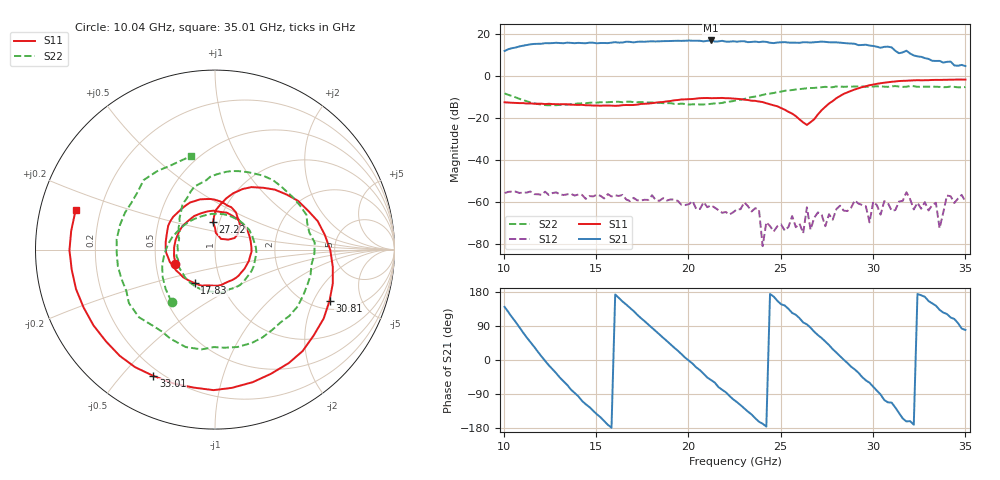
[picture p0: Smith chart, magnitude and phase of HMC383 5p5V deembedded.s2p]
!Hittite Microwave Corporation
!20 Alpha Road
!Chelmsford, MA 01824
!Tel: 978-250-3343
!Fax: 978-250-3373
!Device: HMC383, 12-30 GHz, Driver Amplifier Die
!Misc: Vcc = 5.5V, data includes two K connectors, Room
# MHZ S MA R 50
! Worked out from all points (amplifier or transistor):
!   126 points, 10.04 GHz to 35.01 GHz, reference 50 ohm
!   highest |S21| = 16.7 dB at 21.22 GHz (marker M1)
!   |S21| within 3 dB of that: 10.77 GHz to 30.23 GHz (19.46 GHz wide, 94.9 % of centre)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
!   unconditionally stable (mu >= 1): start of sweep to end of sweep
!   at 14.23 GHz: K = 51.51, MAG = 15.9 dB, |S12| = -56.5 dB
!   at 22.62 GHz: K = 98.47, MAG = 16.8 dB, |S12| = -63.4 dB
!   at 35.01 GHz: K = 71.20, MAG = 10.6 dB, |S12| = -59.7 dB
!   S11 on the Smith chart (normalised r, x): 10.04 GHz: 0.63, -0.11; 17.83 GHz: 0.75, -0.29; 27.22 GHz: 0.94, +0.29; 30.81 GHz: 2.41, -2.69; 33.01 GHz: 0.17, -0.61; 35.01 GHz: 0.11, +0.14
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10037.5  0.234 -160.2  3.865 140.2  0.00165 -18.5  0.379 -129.7
11036.25  0.224 144.4  5.151 72.7  0.001691 -26.9  0.264 173.7
12234.75  0.212 81.7  5.917 -2.4  0.001775 -47.0  0.201 114.7
13433.25  0.209 28.6  6.084 -65.9  0.00154 -67.1  0.207 58.0
14232.25  0.204 -3.3  5.932 -107.9  0.001493 -75.7  0.221 20.9
16030  0.193 -66.6  6.233 172.9  0.001456 -97.2  0.242 -54.8
17827.75  0.218 -121.0  6.5 93.4  0.001131 -120.4  0.232 -118.6
18427  0.235 -139.1  6.544 67.5  0.001077 -118.1  0.228 -137.1
19825.25  0.275 178.1  6.745 6.0  0.0008596 -144.8  0.213 -175.5
21223.5  0.293 135.4  6.852 -52.9  0.0008431 -146.0  0.215 161.9
22621.75  0.283 95.1  6.408 -111.0  0.0006792 -142.3  0.262 139.0
24219.75  0.222 56.1  6.339 -175.7  0.0003338 -172.0  0.369 108.1
25618  0.126 30.6  6.076 124.2  0.0004711 -36.9  0.457 73.1
26816.5  0.093 87.2  6.224 74.5  0.000429 -97.2  0.513 39.6
27216  0.152 94.0  6.439 58.0  0.000505 -41.9  0.533 27.6
28814  0.437 52.0  5.793 -17.6  0.0007411 -93.6  0.551 -20.8
29613  0.563 22.5  5.433 -53.7  0.0008002 -105.7  0.546 -47.5
30811.5  0.699 -24.1  4.879 -111.8  0.0009469 -113.9  0.543 -90.6
31011.25  0.717 -32.4  4.691 -112.4  0.0006254 -119.4  0.561 -97.7
31810.25  0.759 -65.8  3.922 -162.2  0.001718 -157.4  0.547 -128.8
33008.75  0.783 -116.0  2.499 155.6  0.0006362 85.6  0.548 -178.1
35006.25  0.807 164.3  1.693 79.3  0.001032 58.4  0.538 104.3
